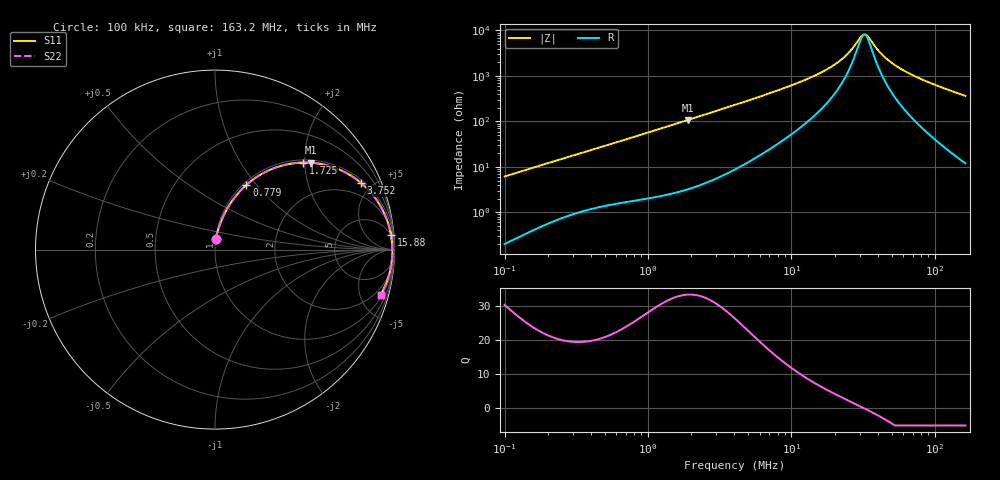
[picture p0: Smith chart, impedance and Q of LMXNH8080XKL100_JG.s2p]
! LMXNH8080XKL100_JG  S-PARAMETER MODEL  ( General Type )
! Model Generated by TAIYO YUDEN Corporation (http://www.ty-top.com)
! Version 1.0
! TAIYO YUDEN Control No. 191025NI43SB-FBB
! Copyright(c) 2019 TAIYO YUDEN CO.,LTD. All Rights Reserved.
! Product Description (link to TY-COMPAS)
! https://ds.yuden.co.jp/TYCOMPAS/or/detail?pn=LMXNH8080XKL100MJG&u=M
! Products Name : Inductors
! Characteristics :
!  Inductance : 10 uH , SRF(min) : 27 MHz , DC Resistance(max) : 0.0429 Ohm
!  Rated Current : Saturation :2400 mA , Temp Rise : 3000 mA
!  Case Size : 8.0 x 8.0 / 0.315 x 0.315 [mm/inch] , Thickness : 3 / 0.118 [mm/inch]
!  (Conditions: Temperature = 25 degC , DC Bias Current/Voltage = 0A / 0V)
! External Node Assignments :
!  1  o---GGG---o  2
! GND o---------o GND
! Frequency Range : 0.1MHz  -  163.203978MHz  [ 402 STEP ]
# MHz S RI R 50
! Freq[MHz].  S11 Real  S11 Imag  S21 Real  S21 Imag  S12 Real  S12 Imag  S22 Real  S22 Imag
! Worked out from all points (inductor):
!   401 points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, 100 kHz to 163.2 MHz, reference 50 ohm
!   read as one part in series: L = 9.73 uH near 103.8 kHz
!   highest Q = 33.4 at 1.893 MHz (marker M1), where L = 9.03 uH
!   self-resonance near 32.06 MHz
!   S11 on the Smith chart (normalised r, x): 100 kHz: 1.00, +0.12; 779 kHz: 1.04, +0.89; 1.725 MHz: 1.06, +1.96; 3.752 MHz: 1.16, +4.29; 15.88 MHz: 5, +23; 163.2 MHz: 1.24, -7.28
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0.1  0.00576 0.061  0.9942 -0.061  0.9942 -0.061  0.00576 0.061
0.345249  0.0488 0.1914  0.9512 -0.1914  0.9512 -0.1914  0.0488 0.1914
0.778992  0.1755 0.361  0.8245 -0.361  0.8245 -0.361  0.1755 0.361
1.191969  0.3203 0.4504  0.6797 -0.4504  0.6797 -0.4504  0.3203 0.4504
1.725446  0.4899 0.4851  0.5101 -0.4851  0.5101 -0.4851  0.4899 0.4851
1.892607  0.5348 0.484  0.4652 -0.484  0.4652 -0.484  0.5348 0.484
3.751786  0.813 0.3722  0.187 -0.3722  0.187 -0.3722  0.813 0.3722
4.115259  0.8385 0.3493  0.1615 -0.3493  0.1615 -0.3493  0.8385 0.3493
6.906982  0.9318 0.2249  0.0682 -0.2249  0.0682 -0.2249  0.9318 0.2249
13.94754  0.9768 0.0997  0.0232 -0.0997  0.0232 -0.0997  0.9768 0.0997
15.87525  0.9803 0.082  0.0197 -0.082  0.0197 -0.082  0.9803 0.082
19.45677  0.9841 0.0565  0.0159 -0.0565  0.0159 -0.0565  0.9841 0.0565
22.98037  0.9861 0.0371  0.0139 -0.0371  0.0139 -0.0371  0.9861 0.0371
26.15651  0.9871 0.0227  0.0129 -0.0227  0.0129 -0.0227  0.9871 0.0227
30.32735  0.9878 0.00668  0.0122 -0.00668  0.0122 -0.00668  0.9878 0.00668
32.05752  0.9879 0.0007  0.0121 -0.0007  0.0121 -0.0007  0.9879 0.0007
33.8864  0.988 -0.00529  0.012 0.00529  0.012 0.00529  0.988 -0.00529
40.77028  0.9877 -0.0255  0.0123 0.0255  0.0123 0.0255  0.9877 -0.0255
48.15376  0.9867 -0.0446  0.0133 0.0446  0.0133 0.0446  0.9867 -0.0446
59.01743  0.9842 -0.0696  0.0158 0.0696  0.0158 0.0696  0.9842 -0.0696
77.88569  0.9778 -0.1083  0.0222 0.1083  0.0222 0.1083  0.9778 -0.1083
163.204  0.9227 -0.2511  0.0773 0.2511  0.0773 0.2511  0.9227 -0.2511
